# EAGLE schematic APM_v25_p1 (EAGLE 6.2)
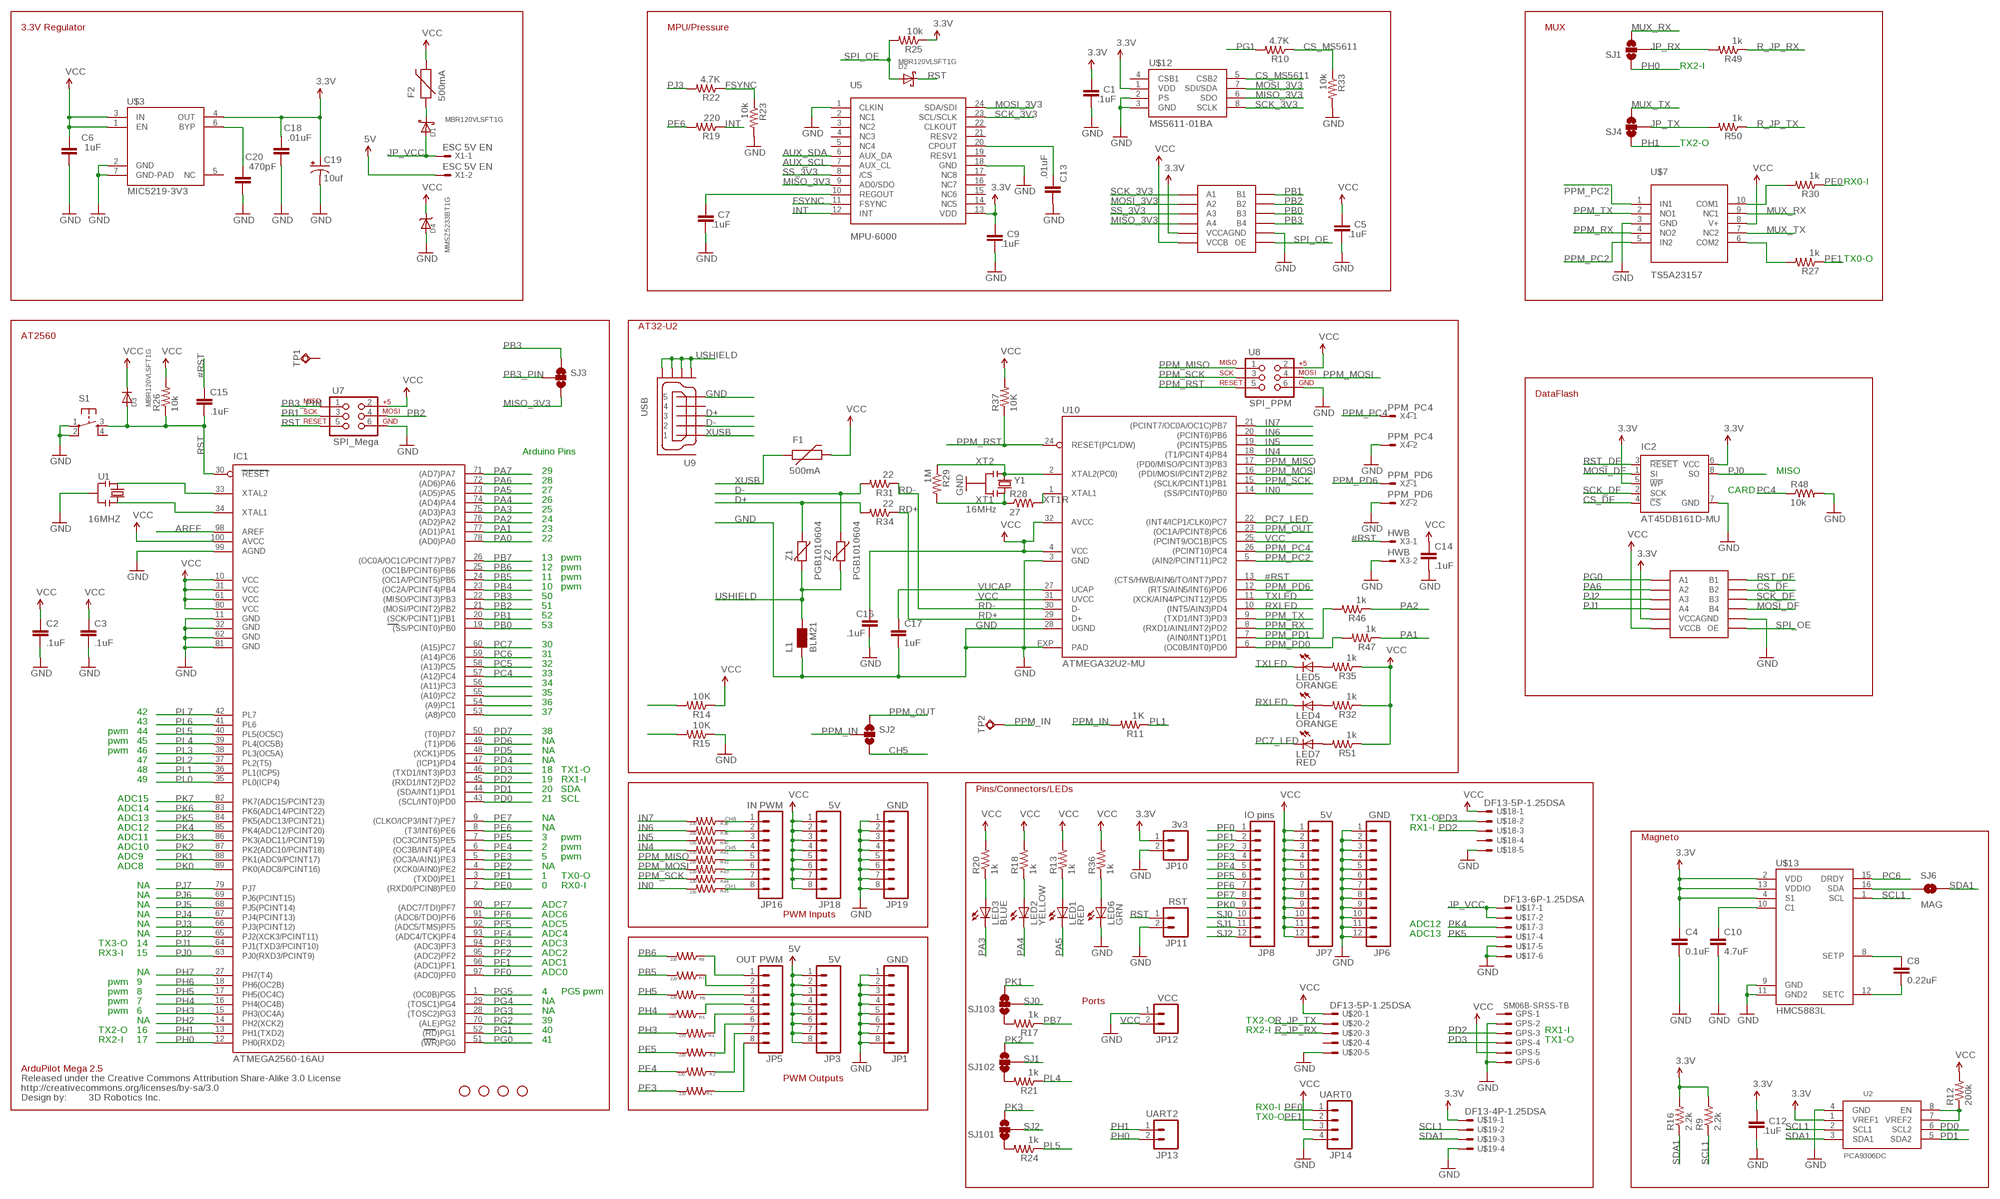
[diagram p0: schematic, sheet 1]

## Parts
C1  .1uF  C-EUC0402  [C0402]
C2  .1uF  CAP0402  [C0402]
C3  .1uF  CAP0402  [C0402]
C4  0.1uF  CAP0402-CAP  [0402-CAP]
C5  .1uF  C-EUC0402  [C0402]
C6  1uF  C-EUC0402  [C0402]
C7  .1uF  C-EUC0402  [C0402]
C8  0.22uF  CAP0402-CAP  [0402-CAP]
C9  .1uF  C-EUC0402  [C0402]
C10  4.7uF  CAP1206  [1206]
C12  .1uF  C-EUC0402  [C0402]
C13  .01uF  C-EUC0402  [C0402]
C14  .1uF  CAP0402  [C0402]
C15  .1uF  CAP0402  [C0402]
C16  .1uF  CAP0402-CAP  [0402-CAP]
C17  1uF  CAP0402-CAP  [0402-CAP]
C18  .01uF  C-EUC0402  [C0402]
C19  10uf  CAP_POL1206  [EIA3216]
C20  470pF  C-EUC0402  [C0402]
D1  MBR120VLSFT1G  DIODESOD-123  [SOD-123]
D2  MBR120VLSFT1G  DIODESOD-123  [SOD-123]
D3  MBR120VLSFT1G  DIODESOD-123  [SOD-123]
D4  MMSZ5233BT1G  DIODESOD-123  [SOD-123]
F1  500mA  PTCSMD  [PTC-1206]
F2  500mA  PTCSMD  [PTC-1206]
GPS  SM06B-SRSS-TB  [SM06B-SRSS-TB]
IC1  ATMEGA2560-16AU  ATMEGA1280-16AU  [TQFP100]
IC2  AT45DB161D-MU  AT45DB161D-MU-NOPAD  [VDFN-8-NO-BOTTOM-PAD]
JP1  GND  M08  [1X08]
JP3  5V  M08  [1X08]
JP5  OUT PWM  M08  [1X08]
JP6  GND  M12PTH  [1X12]
JP7  5V  M12PTH  [1X12]
JP8  IO pins  M12PTH  [1X12]
JP10  3v3  M02PTH  [1X02]
JP11  RST  M02PTH  [1X02]
JP12  VCC  M02PTH  [1X02]
JP13  UART2  M02PTH  [1X02]
JP14  UART0  M04PTH  [1X04]
JP16  IN PWM  M08  [1X08]
JP18  5V  M08  [1X08]
JP19  GND  M08  [1X08]
L1  BLM21  WE-CBF_0805  [0805]
LED1  RED  LED0603  [LED-0603]
LED2  YELLOW  LED0603  [LED-0603]
LED3  BLUE  LED0603  [LED-0603]
LED4  ORANGE  LED0603  [LED-0603]
LED5  ORANGE  LED0603  [LED-0603]
LED6  GRN  LED0603  [LED-0603]
LED7  RED  LED0603  [LED-0603]
R1  220  RESISTOR0402  [C0402]
R2  220  RESISTOR0402  [C0402]
R3  220  RESISTOR0402  [C0402]
R4  220  RESISTOR0402  [C0402]
R5  220  RESISTOR0402  [C0402]
R6  220  RESISTOR0402  [C0402]
R7  220  RESISTOR0402  [C0402]
R8  220  RESISTOR0402  [C0402]
R9  2.2k  RESISTOR0402  [C0402]
R10  4.7K  RESISTOR0402  [C0402]
R11  1K  RESISTOR0402  [C0402]
R12  200k  RESISTOR0402  [C0402]
R13  1k  RESISTOR0402  [C0402]
R14  10K  RESISTOR0402-RES  [0402-RES]
R15  10K  RESISTOR0402-RES  [0402-RES]
R16  2.2k  RESISTOR0402  [C0402]
R17  1k  RESISTOR0402  [C0402]
R18  1k  RESISTOR0402  [C0402]
R19  220  RESISTOR0402  [C0402]
R20  1k  RESISTOR0402  [C0402]
R21  1k  RESISTOR0402  [C0402]
R22  4.7K  RESISTOR0402  [C0402]
R23  10k  RESISTOR0402  [C0402]
R24  1k  RESISTOR0402  [C0402]
R25  10k  RESISTOR0402  [C0402]
R26  10k  RESISTOR0402  [C0402]
R27  1k  RESISTOR0402-RES  [0402-RES]
R28  27  RESISTOR0402-RES  [0402-RES]
R29  1M  RESISTOR0402-RES  [0402-RES]
R30  1k  RESISTOR0402-RES  [0402-RES]
R31  22  RESISTOR0402-RES  [0402-RES]
R32  1k  RESISTOR0402-RES  [0402-RES]
R33  10k  RESISTOR0402  [C0402]
R34  22  RESISTOR0402-RES  [0402-RES]
R35  1k  RESISTOR0402-RES  [0402-RES]
R36  1k  RESISTOR0402  [C0402]
R37  10K  RESISTOR0402-RES  [0402-RES]
R38  220  RESISTOR0402  [C0402]
R39  220  RESISTOR0402  [C0402]
R40  220  RESISTOR0402  [C0402]
R41  220  RESISTOR0402  [C0402]
R42  220  RESISTOR0402  [C0402]
R43  220  RESISTOR0402  [C0402]
R44  220  RESISTOR0402  [C0402]
R45  220  RESISTOR0402  [C0402]
R46  1k  RESISTOR0402-RES  [0402-RES]
R47  1k  RESISTOR0402-RES  [0402-RES]
R48  10k  RESISTOR0402  [C0402]
R49  1k  RESISTOR0402-RES  [0402-RES]
R50  1k  RESISTOR0402-RES  [0402-RES]
R51  1k  RESISTOR0402-RES  [0402-RES]
S1  TAC_SWITCHSMD  [TACTILE_SWITCH_SMD]
SJ1  SOLDERJUMPER_2WAYT  [SJ_2]
SJ2  SOLDERJUMPER_2WAYT  [SJ_2]
SJ3  SOLDERJUMPER_2WAYT  [SJ_2]
SJ4  SOLDERJUMPER_2WAYT  [SJ_2]
SJ6  MAG  SOLDERJUMPERTRACE  [SJ_2S-TRACE]
SJ101  SOLDERJUMPER_2WAYS  [SJ_3]
SJ102  SOLDERJUMPER_2WAYS  [SJ_3]
SJ103  SOLDERJUMPER_2WAYS  [SJ_3]
TP1  TPSQTP10SQ  [TP10SQ]
TP2  TPSQTP10SQ  [TP10SQ]
U1  16MHZ  RESONATORSMD  [RESONATOR-SMD]
U2  PCA9306DC  [VSSOP8]
U5  MPU-6000  MPU-3000  [QFN-24]
U7  SPI_Mega  AVR_SPI_PRG_6NS  [2X3-NS]
U8  SPI_PPM  AVR_SPI_PRG_6NS  [2X3-NS]
U9  USB  MOLEX_MICRO_USB_AB_BOTTOM_MOUNT  [MOLEX_MICRO_USB_AB_BOTTOM_MOUNT]
U10  ATMEGA32U2-MU  ATMEGA8U2-MU  [QFN32]
U$1  STAND-OFF  [STAND-OFF]
U$2  STAND-OFF  [STAND-OFF]
U$3  MIC5219-3V3  MIC5219  [MLF-6]
U$4  STAND-OFF  [STAND-OFF]
U$5  STAND-OFF  [STAND-OFF]
U$6  CREATIVE_COMMONS  [CREATIVE_COMMONS]
U$7  TS5A23157  [MSOP10]
U$12  MS5611-01BA  [MS5611-01BA]
U$13  HMC5883L  [LPCC16]
U$14  TS  BT3412UQFN  [UQFN-12]
U$15  QFN  BT3412UQFN  [UQFN-12]
U$17  DF13-6P-1.25DSA  [DF13-6P-1.25DSA]
U$18  DF13-5P-1.25DSA  [DF13-5P-1.25DSA]
U$19  DF13-4P-1.25DSA  [DF13-4P-1.25DSA]
U$20  DF13-5P-1.25DSA  [DF13-5P-1.25DSA]
X1  ESC 5V EN  87758-0216  [87758-0216]
X2  PPM_PD6  87758-0216  [87758-0216]
X3  HWB  87758-0216  [87758-0216]
X4  PPM_PC4  87758-0216  [87758-0216]
Y1  16MHz  RESONATORMU  [RESONATOR]
Z1  PGB1010604  VARISTORCN0603  [CT/CN0603]
Z2  PGB1010604  VARISTORCN0603  [CT/CN0603]

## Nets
3.3V: C1.2 C4.1 C9.2 C12.2 C18.2 C19.A(+) IC2.5(!WP) IC2.6(VCC) JP10.1 R9.2 R16.2 R25.1 U2.1(VREF1) U5.13(VDD) U$3.4(OUT) U$12.1(VDD) U$13.2(VDD) U$13.4(S1) U$13.13(VDDIO) U$14.1(VCCA) U$15.1(VCCA) U$19.1
5V: JP3.1 JP3.2 JP3.3 JP3.4 JP3.5 JP3.6 JP3.7 JP3.8 X1.2
#RST: C15.1 U10.13((CTS/HWB/AIN6/TO/INT7)PD7) X3.1
AREF: IC1.98(AREF)
AUX_SCL: U5.7(AUX_CL)
AUX_SDA: U5.6(AUX_DA)
CH1: JP16.8 R45.1
CH5: JP16.4 R41.1 SJ2.3
CH8: JP16.1 R38.1
CS_DF: IC2.4(!CS) U$15.9(B2)
CS_MS5611: R10.1 R33.1 U$12.5(CSB2)
D+: R34.2 U9.3 Z1.1
D-: R31.2 U9.2 Z2.1
FSYNC: R22.1 R23.1 U5.11(FSYNC)
GND: C1.1 C2.2 C3.2 C4.2 C5.1 C6.1 C7.1 C9.1 C10.2 C12.1 C13.1 C14.2 C16.2 C17.2 C18.1 C19.C(-) C20.1 D4.A GPS.2 GPS.6 IC1.11(GND) IC1.32(GND1) IC1.62(GND2) IC1.81(GND3) IC1.99(AGND) IC2.7(GND) JP1.1 JP1.2 JP1.3 JP1.4 JP1.5 JP1.6 JP1.7 JP1.8 JP6.1 JP6.2 JP6.3 JP6.4 JP6.5 JP6.6 JP6.7 JP6.8 JP6.9 JP6.10 JP6.11 JP6.12 JP10.2 JP11.2 JP12.1 JP14.4 JP19.1 JP19.2 JP19.3 JP19.4 JP19.5 JP19.6 JP19.7 JP19.8 L1.1 LED6.C R15.1 R23.2 R33.2 R48.2 S1.1 S1.2 U1.2 U2.4(GND) U5.1(CLKIN) U5.18(GND) U7.6 U8.6 U9.5 U10.3(GND) U10.28(UGND) U10.EXP(PAD) U$3.2(GND) U$3.7(GND-PAD) U$7.3(GND) U$12.2(PS) U$12.3(GND) U$13.9(GND) U$13.11(GND2) U$14.6(GND) U$15.6(GND) U$17.5 U$17.6 U$18.5 U$19.4 U$20.5 X2.2 X3.2 X4.2 Y1.2
HI: IC1.53((A8)PC0) IC1.54((A9)PC1) IC1.55((A10)PC2) IC1.56((A11)PC3) R14.2
IN0: R45.2 U10.14((SS/PCINT0)PB0)
IN4: R41.2 U10.18((T1/PCINT4)PB4)
IN5: R40.2 U10.19((PCINT5)PB5)
IN6: R39.2 U10.20((PCINT6)PB6)
IN7: R38.2 U10.21((PCINT7/OC0A/OC1C)PB7)
INT: R19.1 U5.12(INT)
JP_RX: R49.2 SJ1.2
JP_TX: R50.2 SJ4.2
JP_VCC: D1.A U$17.1 U$17.2 X1.1
LO: R15.2
MISO_3V3: SJ3.3 U5.9(AD0/SDO) U$12.6(SDO) U$14.5(A4)
MOSI_3V3: U5.24(SDA/SDI) U$12.7(SDI/SDA) U$14.3(A2)
MOSI_DF: IC2.1(SI) U$15.7(B4)
MUX_RX: SJ1.3 U$7.9(NC1)
MUX_TX: SJ4.3 U$7.7(NC2)
N$1: LED6.A R36.1
N$2: C13.2 U5.20(CPOUT)
N$3: C7.2 U5.10(REGOUT)
N$4: C20.2 U$3.6(BYP)
N$5: D1.C F2.1
N$7: C10.1 U$13.10(C1)
N$8: JP5.5 R4.1
N$9: JP5.6 R3.1
N$10: JP5.7 R2.1
N$11: JP5.8 R1.1
N$12: R12.1 U2.7(VREF2) U2.8(EN)
N$13: JP5.4 R5.1
N$14: JP5.3 R6.1
N$15: JP5.2 R7.1
N$16: JP5.1 R8.1
N$18: LED7.A R51.2
N$19: JP16.2 R39.1
N$20: JP16.3 R40.1
N$22: JP16.5 R42.1
N$23: JP16.6 R43.1
N$24: JP16.7 R44.1
N$25: SJ6.1 U$13.16(SDA)
N$26: C8.1 U$13.8(SETP)
N$27: C8.2 U$13.12(SETC)
N$28: LED1.A R13.1
N$29: LED5.A R35.2
N$30: LED4.A R32.2
N$31: LED2.A R18.1
N$32: R30.2 U$7.10(COM1)
N$33: R27.2 U$7.6(COM2)
N$34: LED3.A R20.1
N$36: R17.2 SJ103.1
N$38: R24.2 SJ101.1
N$39: R21.2 SJ102.1
N$56: IC1.34(XTAL1) U1.3
N$89: IC1.33(XTAL2) U1.1
PA0: IC1.78((AD0)PA0)
PA1: IC1.77((AD1)PA1) R47.1
PA2: IC1.76((AD2)PA2) R46.1
PA3: IC1.75((AD3)PA3) LED3.C
PA4: IC1.74((AD4)PA4) LED2.C
PA5: IC1.73((AD5)PA5) LED1.C
PA6: IC1.72((AD6)PA6) U$15.3(A2)
PA7: IC1.71((AD7)PA7)
PB0: IC1.19((SS/PCINT0)PB0) U$14.8(B3)
PB1: IC1.20((SCK/PCINT1)PB1) U7.3 U$14.10(B1)
PB2: IC1.21((MOSI/PCINT2)PB2) U7.4 U$14.9(B2)
PB3: IC1.22((MISO/PCINT3)PB3) SJ3.1 U$14.7(B4)
PB3_PIN: SJ3.2 U7.1
PB4: IC1.23((OC2A/PCINT4)PB4)
PB5: IC1.24((OC1A/PCINT5)PB5) R7.2
PB6: IC1.25((OC1B/PCINT6)PB6) R8.2
PB7: IC1.26((OC0A/OC1C/PCINT7)PB7) R17.1
PC4: IC1.57((A12)PC4) R48.1
PC5: IC1.58((A13)PC5)
PC6: IC1.59((A14)PC6) U$13.15(DRDY)
PC7: IC1.60((A15)PC7)
PC7_LED: LED7.C U10.22((INT4/ICP1/CLK0)PC7)
PD0: IC1.43((SCL/INT0)PD0) U2.6(SCL2)
PD1: IC1.44((SDA/INT1)PD1) U2.5(SDA2)
PD2: GPS.3 IC1.45((RXD1/INT2)PD2) U$18.3
PD3: GPS.4 IC1.46((TXD1/INT3)PD3) U$18.2
PD4: IC1.47((ICP1)PD4)
PD5: IC1.48((XCK1)PD5)
PD6: IC1.49((T1)PD6)
PD7: IC1.50((T0)PD7)
PE0: IC1.2((RXD0/PCIN8)PE0) JP14.1 R30.1
PE1: IC1.3((TXD0)PE1) JP14.2 R27.1
PE2: IC1.4((XCK0/AIN0)PE2)
PE3: IC1.5((OC3A/AIN1)PE3) R1.2
PE4: IC1.6((OC3B/INT4)PE4) R2.2
PE5: IC1.7((OC3C/INT5)PE5) R3.2
PE6: IC1.8((T3/INT6)PE6) R19.2
PE7: IC1.9((CLKO/ICP3/INT7)PE7)
PF0: IC1.97((ADC0)PF0) JP8.1
PF1: IC1.96((ADC1)PF1) JP8.2
PF2: IC1.95((ADC2)PF2) JP8.3
PF3: IC1.94((ADC3)PF3) JP8.4
PF4: IC1.93((ADC4/TCK)PF4) JP8.5
PF5: IC1.92((ADC5/TMS)PF5) JP8.6
PF6: IC1.91((ADC6/TDO)PF6) JP8.7
PF7: IC1.90((ADC7/TDI)PF7) JP8.8
PG0: IC1.51((WR)PG0) U$15.2(A1)
PG1: IC1.52((RD)PG1) R10.2
PG2: IC1.70((ALE)PG2)
PG3: IC1.28((TOSC2)PG3)
PG4: IC1.29((TOSC1)PG4)
PG5: IC1.1((OC0B)PG5)
PH0: IC1.12(PH0(RXD2)) JP13.2 SJ1.1
PH1: IC1.13(PH1(TXD2)) JP13.1 SJ4.1
PH2: IC1.14(PH2(XCK2))
PH3: IC1.15(PH3(OC4A)) R4.2
PH4: IC1.16(PH4(OC4B)) R5.2
PH5: IC1.17(PH5(OC4C)) R6.2
PH6: IC1.18(PH6(OC2B))
PH7: IC1.27(PH7(T4))
PJ0: IC1.63(PJ0(RXD3/PCINT9)) IC2.8(SO)
PJ1: IC1.64(PJ1(TXD3/PCINT10)) U$15.5(A4)
PJ2: IC1.65(PJ2(XCK3/PCINT11)) U$15.4(A3)
PJ3: IC1.66(PJ3(PCINT12)) R22.2
PJ4: IC1.67(PJ4(PCINT13))
PJ5: IC1.68(PJ5(PCINT14))
PJ6: IC1.69(PJ6(PCINT15))
PJ7: IC1.79(PJ7)
PK0: IC1.89(PK0(ADC8/PCINT16)) JP8.9
PK1: IC1.88(PK1(ADC9/PCINT17)) SJ103.3
PK2: IC1.87(PK2(ADC10/PCINT18)) SJ102.3
PK3: IC1.86(PK3(ADC11/PCINT19)) SJ101.3
PK4: IC1.85(PK4(ADC12/PCINT20)) U$17.3
PK5: IC1.84(PK5(ADC13/PCINT21)) U$17.4
PK6: IC1.83(PK6(ADC14/PCINT22))
PK7: IC1.82(PK7(ADC15/PCINT23))
PL0: IC1.35(PL0(ICP4))
PL1: IC1.36(PL1(ICP5)) R11.1
PL2: IC1.37(PL2(T5))
PL3: IC1.38(PL3(OC5A))
PL4: IC1.39(PL4(OC5B)) R21.1
PL5: IC1.40(PL5(OC5C)) R24.1
PL6: IC1.41(PL6)
PL7: IC1.42(PL7)
PPM_IN: R11.2 SJ2.2 TP2.TP
PPM_MISO: R42.2 U8.1 U10.17((PD0/MISO/PCINT3)PB3)
PPM_MOSI: R43.2 U8.4 U10.16((PDI/MOSI/PCINT2)PB2)
PPM_OUT: SJ2.1 U10.23((OC1A/PCINT8)PC6)
PPM_PC2: U10.5((AIN2/PCINT11)PC2) U$7.1(IN1) U$7.5(IN2)
PPM_PC4: U10.26((PCINT10)PC4) X4.1
PPM_PD0: R47.2 U10.6((OC0B/INT0)PD0)
PPM_PD1: R46.2 U10.7((AIN0/INT1)PD1)
PPM_PD6: U10.12((RTS/AIN5/INT6)PD6) X2.1
PPM_RST: R37.1 U8.5 U10.24(RESET(PC1/DW))
PPM_RX: U10.8((RXD1/AIN1/INT2)PD2) U$7.4(NO2)
PPM_SCK: R44.2 U8.3 U10.15((SCLK/PCINT1)PB1)
PPM_TX: U10.9((TXD1/INT3)PD3) U$7.2(NO1)
R_JP_RX: R49.1 U$20.3
R_JP_TX: R50.1 U$20.2
RD+: R34.1 U10.29(D+)
RD-: R31.1 U10.30(D-)
RST: C15.2 D2.C D3.A IC1.30(RESET) JP11.1 R26.1 S1.3 U7.5
RST_DF: IC2.3(!RESET) U$15.10(B1)
RXLED: LED4.C U10.10((INT5/AIN3)PD4)
SCK_3V3: U5.23(SCL/SCLK) U$12.8(SCLK) U$14.2(A1)
SCK_DF: IC2.2(SCK) U$15.8(B3)
SCL1: R9.1 U2.2(SCL1) U$13.1(SCL) U$19.2
SDA1: R16.1 SJ6.2 U2.3(SDA1) U$19.3
SJ0: JP8.10 SJ103.2
SJ1: JP8.11 SJ102.2
SJ2: JP8.12 SJ101.2
SPI_OE: D2.A R25.2 U$14.12(OE) U$15.12(OE)
SS_3V3: U5.8(/CS) U$14.4(A3)
TXLED: LED5.C U10.11((XCK/AIN4/PCINT12)PD5)
USHIELD: L1.2 U9.GND1 U9.GND2 U9.GND3 U9.GND4 Z1.2 Z2.2
VCC: C2.1 C3.1 C5.2 C6.2 C14.1 C16.1 D3.C D4.C F1.2 F2.2 GPS.5 IC1.10(VCC) IC1.31(VCC1) IC1.61(VCC2) IC1.80(VCC3) IC1.100(AVCC) JP7.1 JP7.2 JP7.3 JP7.4 JP7.5 JP7.6 JP7.7 JP7.8 JP7.9 JP7.10 JP7.11 JP7.12 JP12.2 JP14.3 JP18.1 JP18.2 JP18.3 JP18.4 JP18.5 JP18.6 JP18.7 JP18.8 R12.2 R13.2 R14.1 R18.2 R20.2 R26.2 R32.1 R35.1 R36.2 R37.2 R51.1 U7.2 U8.2 U10.4(VCC) U10.25((PCINT9/OC1B)PC5) U10.31(UVCC) U10.32(AVCC) U$3.1(EN) U$3.3(IN) U$7.8(V+) U$14.11(VCCB) U$15.11(VCCB) U$18.1 U$20.1
VUCAP: C17.1 U10.27(UCAP)
XT1: R28.1 R29.2 Y1.3
XT1R: R28.2 U10.1(XTAL1)
XT2: R29.1 U10.2(XTAL2(PC0)) Y1.1
XUSB: F1.1 U9.1
Unconnected: GPS.1 S1.4 TP1.TP U5.2(NC1) U5.3(NC2) U5.4(NC3) U5.5(NC4) U5.14(NC5) U5.15(NC6) U5.16(NC7) U5.17(NC8) U5.19(RESV1) U5.21(RESV2) U5.22(CLKOUT) U9.4 U$3.5(NC) U$12.4(CSB1) U$18.4 U$20.4

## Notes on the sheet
- 3.3V Regulator | MPU/Pressure | MUX
- RX2-I
- TX2-O
- RX0-I
- TX0-O
- AT32-U2
- AT2560
- DataFlash
- Arduino Pins
- 29 | MISO
- 28
- 27 | CARD
- 26
- 25
- 24
- 23
- 22
- 13 | pwm
- 12 | pwm
- 11 | pwm
- 10 | pwm
- 50
- 51
- 52
- 53
- 30
- 31
- 32
- 33
- 34
- 35
- 36
- 42 | 37
- 43
- pwm | 44 | 38
- pwm | 45 | NA
- pwm | 46 | NA
- 47 | NA
- 48 | 18 | TX1-O
- 49 | 19 | RX1-I
- 20 | SDA | Pins/Connectors/LEDs
- ADC15 | 21 | SCL
- ADC14
- ADC13 | NA | TX1-O
- ADC12 | NA | RX1-I
- ADC11 | 3 | pwm | Magneto
- ADC10 | 2 | pwm
- ADC9 | 5 | pwm
- ADC8 | NA
- 1 | TX0-O
- NA | 0 | RX0-I
- NA
- NA | ADC7
- NA | ADC6 | PWM Inputs
- NA | ADC5 | ADC12
- NA | ADC4 | ADC13
- TX3-O | 14 | ADC3
- RX3-I | 15 | ADC2
- ADC1
- NA | ADC0
- pwm | 9
- pwm | 8 | 4 | PG5 pwm
- pwm | 7 | NA | Ports
- pwm | 6 | NA
- NA | 39 | TX2-O
- TX2-O | 16 | 40 | RX2-I | RX1-I
- RX2-I | 17 | 41 | TX1-O
- ArduPilot Mega 2.5
- PWM Outputs
- 3D Robotics Inc.
- RX0-I
- TX0-O

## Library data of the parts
C1 C5-C7 C9 C12 C13 C18 C20 = SmartPrj:C-EU: CAPACITOR, European symbol
C2 C3 C14 C15 = DIYdrones3:CAP: Capacitor
C4 C8 C10 C16 C17 = SparkFun:CAP: Capacitor
C19 = SparkFun:CAP_POL: Capacitor Polarized
D1-D4 = adafruit:DIODE: Diode
F1 F2 = SparkFun:PTC: Resettable Fuse PTC
GPS = con-jst2:?M06B-SRSS-TB: Disconnectable Crimp style connector, 1.0mm pitch 6 contacts
IC1 = atmel-2010:ATMEGA*: MICROCONTROLLER 64/128/256 Kbytes FLASH 4 Kbytes EEPROM 8 Kbytes SRAM 86 General Purpose I/O pins 12-channels16-bit PWM 4 x Serial USARTs 16-channels 10-bit A/D
IC2 = 3DRobotics:AT45DB161D: Atmel 16-megabit 2.5V or 2.7V DataFlash The Atmel® AT45DB161D is a 2.5V or 2.7V, serial-interface sequential access Flash memory ideally suited for a wide variety of digital voice-, image-, program code- and data-storage applications. The AT45DB161D supports Atmel RapidS? serial interface for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; DATASHEET: http://www.atmel.com/dyn/resources/prod_documents/doc3500.pdf; LINK: http://www.atmel.com/dyn/products/product_card.asp?part_id=3772; MFGPN: AT45DB161D-MU
JP1 JP3 JP5 JP16 JP18 JP19 = SparkFunv2:M08: Header 8 Standard 8-pin 0.1" header. Use with straight break away headers (SKU : PRT-00116), right angle break away headers (PRT-00553), swiss pins (PRT-00743), machine pins (PRT-00117), and female headers (PRT-00115).
JP6-JP8 = SparkFun:M12: Header 12 Standard 12-pin 0.1" header. Use with straight break away headers (SKU : PRT-00116), right angle break away headers (PRT-00553), swiss pins (PRT-00743), machine pins (PRT-00117), and female headers (PRT-00115).
JP10-JP13 = SparkFun:M02: Header 2
JP14 = SparkFun:M04: Header 4 Standard 4-pin 0.1" header. Use with straight break away headers (SKU : PRT-00116), right angle break away headers (PRT-00553), swiss pins (PRT-00743), machine pins (PRT-00117), and female headers (PRT-00115). Molex polarized connector foot print use with SKU : PRT-08231 with associated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
L1 = wuerth-elektronik:WE-CBF: SMD EMI Suppression Ferrite Beads
LED1-LED3 LED6 = DIYdrones3:LED: LEDs
LED4 LED5 LED7 = SparkFun:LED: LEDs
R1-R13 R16-R26 R33 R36 R38-R45 R48 = DIYdrones3:RESISTOR: Resistor
R14 R15 R27-R32 R34 R35 R37 R46 R47 R49-R51 = SparkFun:RESISTOR: Resistor
S1 = DIYdrones3:TAC_SWITCH: Momentary Switch Button commonly used for reset or general input. Spark Fun Electronics SKU : COM-00097
SJ1-SJ4 SJ101-SJ103 = SparkFun:SOLDERJUMPER_2WAY: Solder Jumper 2 way solder jumper
SJ6 = SparkFun:SOLDERJUMPER: Solder Jumper
TP1 TP2 = testpad:TPSQ: Test pad
U1 = DIYdrones3:RESONATOR: Resonator Small SMD resonator. This is the itty bitty 10/20MHz resonators with built in caps. CSTCE10M0G55 and CSTCE20M0V53. Footprint has been reviewed closely but hasn't been tested yet.
U2 = DIYdrones_082610:PCA9306DC
U5 = 3DRobotics_Master_Library:MPU-3000: Invensense MPU-3000 Motion Processing Unit The MPU-30X0 Motion Processing Unit (MPU?) is the world?s first motion processing solution with integrated 6-axis sensor fusion for smart phone applications. The MPU-30X0 has an embedded 3- axis gyroscope and Digital Motion Processor? (DMP) hardware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; DATASHEET: http://invensense.com/mems/gyro/documents/PS-MPU-3000A-00_v2.6.pdf; LINK: http://www.invensense.com/mems/gyro/mpu3000.html; MFGPN: MPU-3000
U7 U8 = SparkFunv2:AVR_SPI_PRG_6: AVR ISP 6 Pin This is the reduced ISP connector for AVR programming. Common on Arduino. This footprint will take up less PCB space and can be used with a 10-pin to 6-pin adapter such as SKU: BOB-08508
U9 = 3DRobotics:MOLEX_MICRO_USB_AB_BOTTOM_MOUNT: Molex Micro USB AB Bottom Mount Receptacle; DATASHEET: http://www.molex.com/pdm_docs/sd/475890001_sd.pdf; LINK: http://www.molex.com/molex/products/datasheet.jsp?part=active/0475890001_IO_CONNECTORS.xml&channel=Products&Lang=en-US; MFGPN: 47589-0001
U10 = atmel:ATMEGA8U2-MU
U$1 U$2 U$4 U$5 = DIYdrones3:STAND-OFF: Stand Off
U$3 = 3DRobotics:MIC5219: Micrel MIC5219 500mA peak output LDO regulator The MIC5219 is an efficient linear voltage regulator with high peak output current capability, very-low-dropout voltage, and better than 1% output voltage accuracy. Dropout is typically 10mV at light loads and less than 500mV at full load. The MIC5219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; DATASHEET: http://www.micrel.com/_PDF/mic5219.pdf; LINK: http://www.micrel.com/page.do?page=/product-info/products/mic5219.shtml; MFGPN: MIC5219
U$6 = SparkFun:CREATIVE_COMMONS
U$7 = 3DRobotics:TS5A23157: TS5A23157 Dual 10-Ohm SPDT Analog Switch The TS5A23157 is a dual single-pole double-throw (SPDT) analog switch designed to operate from 1.65 V to 5.5 V. This device can handle both digital and analog signals. Signals up to 5.5 V (peak) can be transmitted in either direction.; DATASHEET: http://focus.ti.com/lit/ds/symlink/ts5a23157.pdf; LINK: http://focus.ti.com/docs/prod/folders/print/ts5a23157.html; MFGPN: TS5A23157DGSR
U$12 = 3DRobotics:MS5611-01BA: MS5611-01BA The MS5611-01BA is a new generation of high resolution altimeter sensors from MEAS Switzerland with SPI and I 2 C bus interface. It is optimized for altimeters and variometers with an altitude resolution of 10 cm. The sensor module includes a high linearity pressure sensor and an ultra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; DATASHEET: http://www.meas-spec.com/downloads/MS5611-01BA01.pdf; LINK: http://www.meas-spec.com/product/t_product.aspx?id=8503#; MFGPN: MS5611-01BA
U$13 = 3DRobotics:HMC5883L: Honeywell HMC5883L 3-axis digital compass IC Successor to the HMC5843.; DATASHEET: http://www.dsscircuits.com/images/datasheets/HMC5883L.pdf; LINK: http://parts.digikey.com/1/parts/2057013-ic-compass-3-axis-i2c-16lcc-smd-hmc5883l-tr.html; MFGPN: HMC5883L-TR
U$14 U$15 = 3DRobotics:BT3412: TI BT3412 4-Bit Bidirectional Voltage-Level Translator with Auto Direction Sensing This 4-bit noninverting translator uses two separate configurable power-supply rails. The A port is designed to track VCCA. VCCA accepts any supply voltage from 1.2 V to 3.6 V. The B port is designed to track VCCB.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
U$17 = pixhawk2:DF13-6P-1.25?
U$18 U$20 = pixhawk2:DF13-5P-1.25?
U$19 = pixhawk2:DF13-4P-1.25?
X1-X4 = con-molex:87758-0216: 2 Pin - 2mm Dual Row Single Wafer, Vertical T/H HDR; MPN: 87758-0216; OC_FARNELL: unknown; OC_NEWARK: 94M1513
Y1 = SmartPrj:RESONATOR
Z1 Z2 = varistor:VARISTOR: VARISTOR

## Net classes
0 default: width 0.178 mm, drill 0.381 mm, clearance 0.178 mm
